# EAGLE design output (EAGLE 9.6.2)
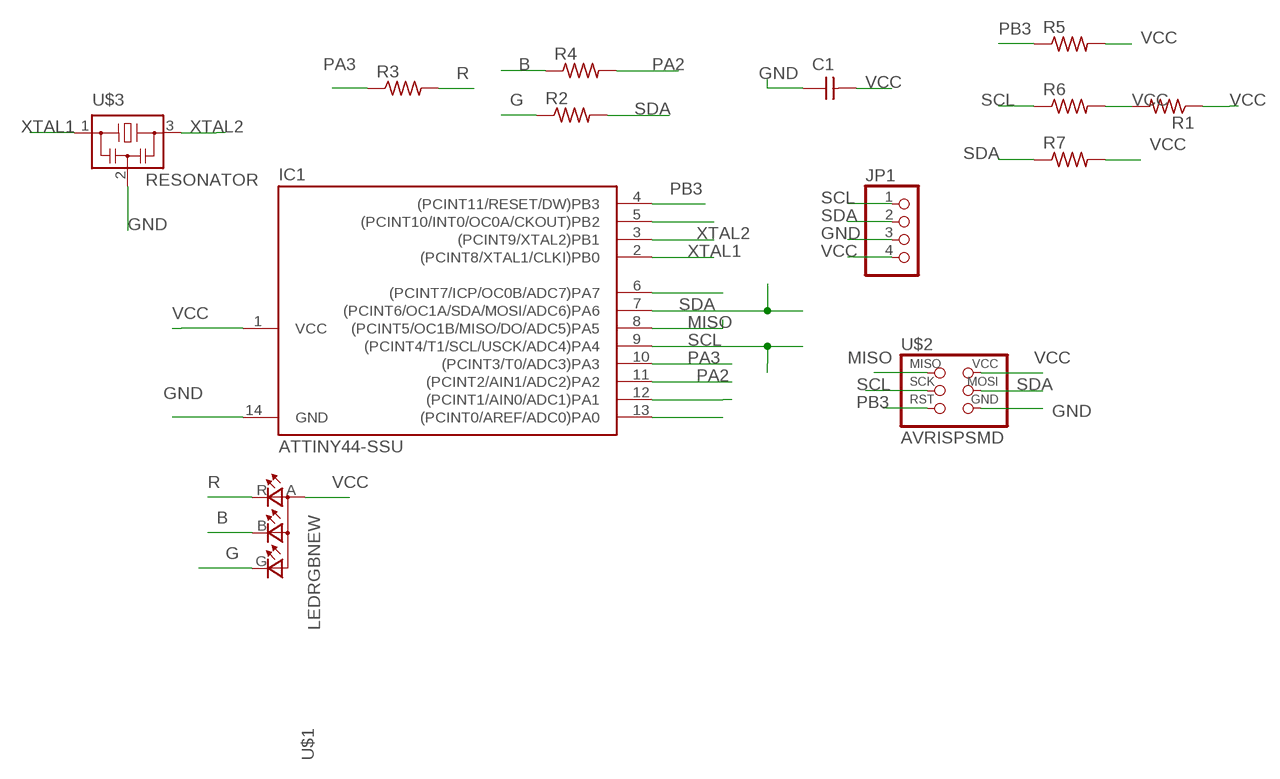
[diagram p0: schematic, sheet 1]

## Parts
C1  CAP-UNPOLARIZED  [C1206]
IC1  ATTINY44-SSU  [SOIC14]
JP1  PINHD-1X4  [1X04]
R1  RES-US1206  [R1206]
R2  RES-US1206  [R1206]
R3  RES-US1206  [R1206]
R4  RES-US1206  [R1206]
R5  RES-US1206  [R1206]
R6  RES-US1206  [R1206]
R7  RES-US1206  [R1206]
U$1  LEDRGBNEW  [P-LCC-4]
U$2  AVRISPSMD  [2X03SMD]
U$3  RESONATOR  [EFOBM]

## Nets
B: R4.1 U$1.B(CBLUE)
G: R2.1 U$1.G(CGREEN)
GND: C1.1 IC1.14(GND) JP1.3 U$2.6(GND) U$3.2
MISO: IC1.8((PCINT5/OC1B/MISO/DO/ADC5)PA5) U$2.1(MISO)
N$30: IC1.5((PCINT10/INT0/OC0A/CKOUT)PB2)
N$33: IC1.6((PCINT7/ICP/OC0B/ADC7)PA7)
N$39: IC1.12((PCINT1/AIN0/ADC1)PA1)
N$40: IC1.13((PCINT0/AREF/ADC0)PA0)
PA2: IC1.11((PCINT2/AIN1/ADC2)PA2) R4.2
PA3: IC1.10((PCINT3/T0/ADC3)PA3) R3.1
PB3: IC1.4((PCINT11/RESET/DW)PB3) R5.1 U$2.5(RST)
R: R3.2 U$1.R(CRED)
SCL: IC1.9((PCINT4/T1/SCL/USCK/ADC4)PA4) JP1.1 R6.1 U$2.3(SCK)
SDA: IC1.7((PCINT6/OC1A/SDA/MOSI/ADC6)PA6) JP1.2 R2.2 R7.1 U$2.4(MOSI)
VCC: C1.2 IC1.1(VCC) JP1.4 R1.1 R1.2 R5.2 R6.2 R7.2 U$1.A(A2) U$2.2(VCC)
XTAL1: IC1.2((PCINT8/XTAL1/CLKI)PB0) U$3.1
XTAL2: IC1.3((PCINT9/XTAL2)PB1) U$3.3

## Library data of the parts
C1 = fab:CAP-UNPOLARIZED
IC1 = fab:ATTINY44
JP1 = pinhead:PINHD-1X4: PIN HEADER
R1-R7 = fab:RES-US: Resistor (US Symbol)
U$1 = fab:LEDRGBNEW
U$2 = fab:AVRISP
U$3 = fab:RESONATOR

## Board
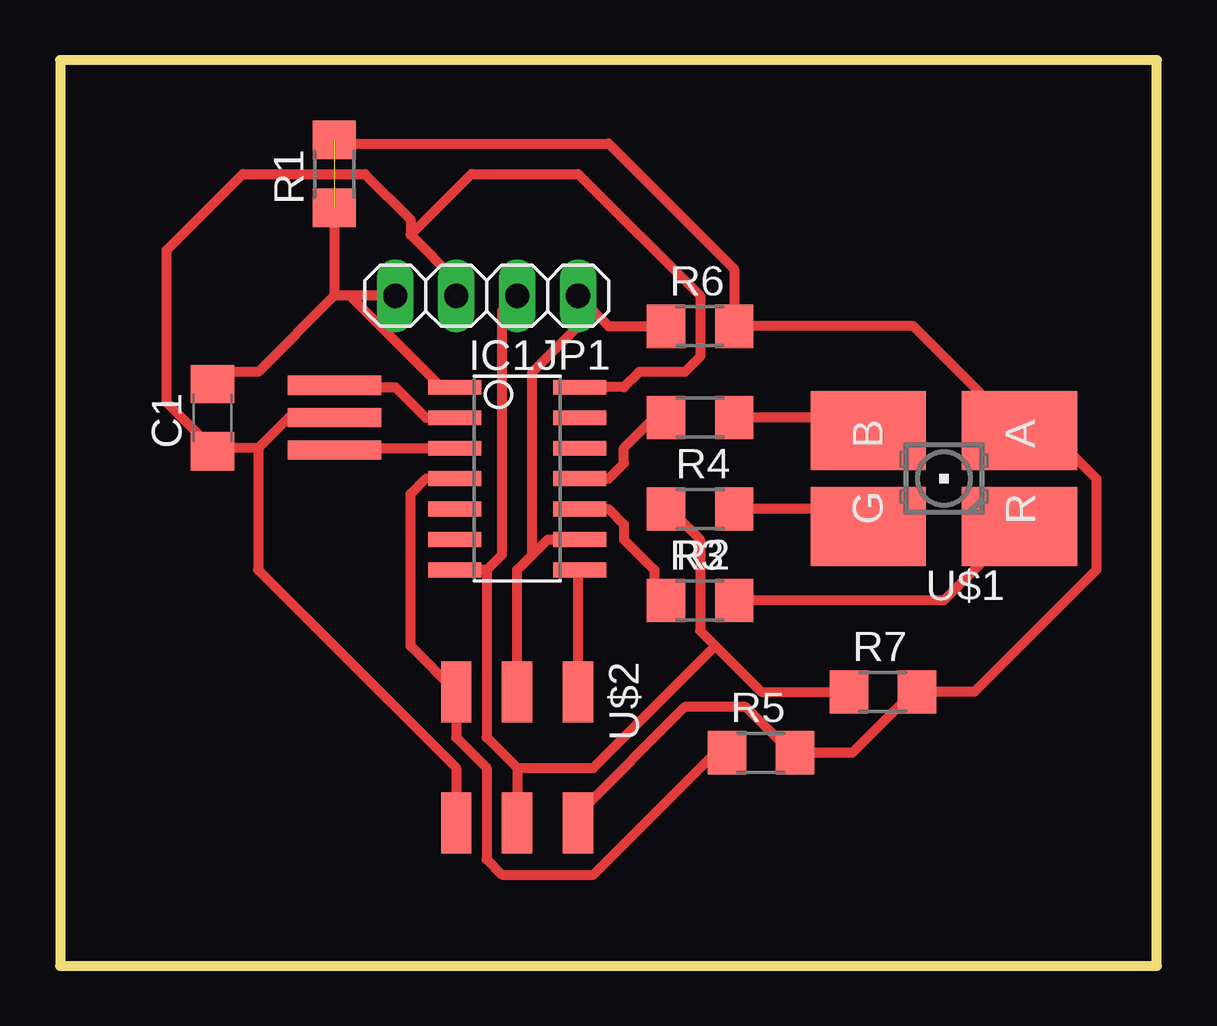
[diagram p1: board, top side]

Size 45.7 x 37.77 mm. Coordinates in mm from the lower left corner, seen from the top.
Outline: 0,0 45.7,0 45.7,37.77 0,37.77 0,0
Copper layers (1*16): Top 0.035mm / dielectric 1.5mm / Bottom 0.035mm
Design rules "default *": minimum track width 16mil, minimum drill 0.35mm, track to track 16mil, track to pad 16mil, pad to pad 16mil, via to via 16mil, smd to smd 16mil, copper to edge 40mil, drill to drill 16mil, minimum pad ring 10mil, minimum via ring 8mil, stop-mask expansion 4mil, vias tented up to drill 0mil, thermal gap 10mil

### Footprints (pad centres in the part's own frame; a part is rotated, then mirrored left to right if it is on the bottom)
C1206 = smd 1.6 x 1.8: 1 -1.4,0; 2 1.4,0
SOIC14 = smd 0.61 x 2.21: 1 -3.81,-2.603; 2 -2.54,-2.603; 3 -1.27,-2.603; 4 0,-2.603; 5 1.27,-2.603; 6 2.54,-2.603; 7 3.81,-2.603; 8 3.81,2.603; 9 2.54,2.603; 10 1.27,2.603; 11 0,2.603; 12 -1.27,2.603; 13 -2.54,2.603; 14 -3.81,2.603
1X04 = drill 1.016 long: 1 -3.81,0; 2 -1.27,0; 3 1.27,0; 4 3.81,0
R1206 = smd 1.6 x 1.803: 1 -1.422,0; 2 1.422,0
P-LCC-4 = smd 3.3 x 4.8: A 2,-3.15; B 2,3.15; G -2,3.15; R -2,-3.15
2X03SMD = smd 2.54 x 1.27: 1 -2.54,2.54; 2 2.92,2.54; 3 -2.54,0; 4 2.92,0; 5 -2.54,-2.54; 6 2.92,-2.54
EFOBM = smd 0.8 x 3.9: 1 -1.35,0; 2 0,0; 3 1.35,0

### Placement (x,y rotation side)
C1  6.35,22.86 90 top
IC1  19.05,20.32 270 top
JP1  17.78,27.94 180 top
R1  11.43,33.02 90 top
R2  26.67,19.05 180 top
R3  26.67,15.24 0 top
R4  26.67,22.86 180 top
R5  29.21,8.89 0 top
R6  26.67,26.67 0 top
R7  34.29,11.43 0 top
U$1  36.83,20.32 90 top
U$2  19.05,8.89 270 top
U$3  11.43,22.86 270 top

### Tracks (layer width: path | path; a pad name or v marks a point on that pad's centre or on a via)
B
  Top 0.406: R4.1 33.66,22.86 U$1.B
G
  Top 0.406: R2.1 33.02,19.05 33.66,18.41 U$1.G
GND
  Top 0.406: IC1.14 23.5,24.13 24.13,24.77 26.04,24.77 26.67,25.4 26.67,27.94 21.59,33.02 17.14,33.02 14.61,30.48 | 8.25,21.59 6.35,21.59 | 8.25,21.59 9.52,22.86 U$3.2 | U$2.6 16.51,8.25 8.25,16.51 8.25,21.59 | 14.61,30.48 16.51,28.58 JP1.3 | 6.35,21.59 4.45,23.49 4.45,29.84 7.62,33.02 12.7,33.02 14.61,31.12 14.61,30.48 | 6.35,21.59 C1.1
MISO
  Top 0.406: U$2.1 21.59,16.51 IC1.8
PA2
  Top 0.406: IC1.11 22.86,20.32 23.5,20.95 23.5,21.59 24.76,22.86 R4.2
PA3
  Top 0.406: IC1.10 22.86,19.05 23.5,18.41 23.5,17.78 24.76,16.51 24.76,15.24 R3.1
PB3
  Top 0.406: R5.1 27.31,8.89 22.22,3.81 18.41,3.81 17.78,4.45 17.78,8.25 16.51,9.52 U$2.5 14.61,13.34 14.61,19.68 15.24,20.32 IC1.4
R
  Top 0.406: R3.2 36.83,15.24 39.37,17.78 U$1.R
SCL
  Top 0.406: R6.1 22.86,26.67 22.22,27.3 | IC1.9 20.32,17.78 19.68,17.14 | 19.68,17.14 19.05,16.51 U$2.3 | 22.22,27.3 19.68,24.77 19.68,17.14 | 22.22,27.3 JP1.1
SDA
  Top 0.406: R7.1 29.21,11.43 27.31,13.34 | 27.31,13.34 26.67,13.97 26.67,17.78 25.4,19.05 R2.2 | 17.78,16.51 IC1.7 | 17.78,16.51 18.41,17.14 18.41,27.3 JP1.2 | 19.05,8.25 U$2.4 | 19.05,8.25 17.78,9.52 17.78,16.51 | 27.31,13.34 22.22,8.25 19.05,8.25
VCC  (1 unrouted)
  Top 0.406: U$2.2 21.59,6.35 26.04,10.8 28.57,10.8 30.48,8.89 R5.2 33.02,8.89 35.56,11.43 R7.2 38.1,11.43 43.18,16.51 43.18,20.32 41.28,22.23 40,22.23 U$1.A 39.37,22.86 35.56,26.67 R6.2 | 11.43,27.94 8.25,24.77 6.35,24.77 C1.2 | JP1.4 12.07,27.94 | 12.07,27.94 11.43,27.94 | 12.07,27.94 15.88,24.13 IC1.1 | R1.1 11.43,27.94 | 27.94,26.67 R6.2 | R1.2 11.58,34.29 22.86,34.29 28.09,29.06 R6.2
XTAL1
  Top 0.406: IC1.2 15.24,22.86 13.97,24.13 11.43,24.13 U$3.1
XTAL2
  Top 0.406: IC1.3 11.43,21.59 U$3.3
